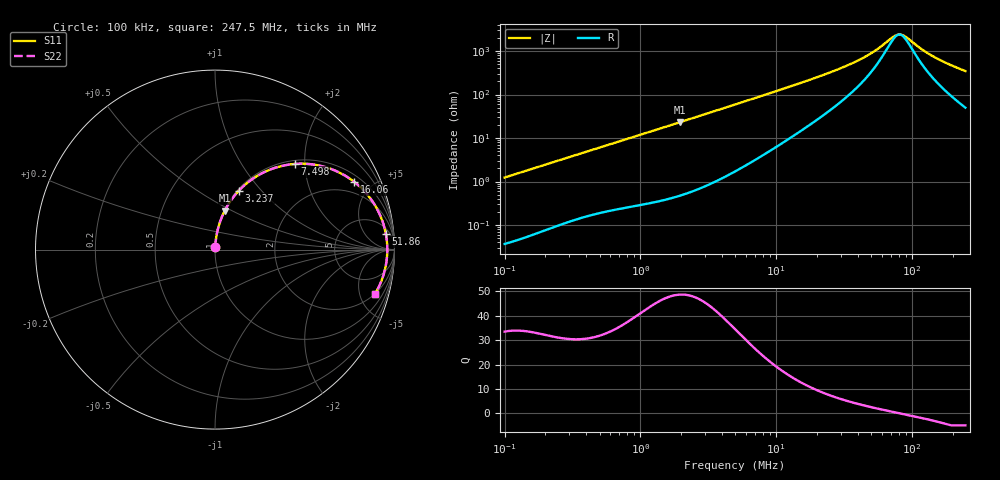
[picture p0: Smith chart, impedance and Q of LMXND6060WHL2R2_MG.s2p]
! LMXND6060WHL2R2_MG  S-PARAMETER MODEL  ( General Type )
! Model Generated by TAIYO YUDEN Corporation (http://www.ty-top.com)
! Version 1.0
! TAIYO YUDEN Control No. 191025NI43SB-FBB
! Copyright(c) 2019 TAIYO YUDEN CO.,LTD. All Rights Reserved.
! Product Description (link to TY-COMPAS)
! https://ds.yuden.co.jp/TYCOMPAS/or/detail?pn=LMXND6060WHL2R2NMG&u=M
! Products Name : Inductors
! Characteristics :
!  Inductance : 2.2 uH , SRF(min) : 68 MHz , DC Resistance(max) : 0.026 Ohm
!  Rated Current : Saturation :4200 mA , Temp Rise : 3700 mA
!  Case Size : 6.0 x 6.0 / 0.236 x 0.236 [mm/inch] , Thickness : 2.8 / 0.11 [mm/inch]
!  (Conditions: Temperature = 25 degC , DC Bias Current/Voltage = 0A / 0V)
! External Node Assignments :
!  1  o---GGG---o  2
! GND o---------o GND
! Frequency Range : 0.1MHz  -  247.502633MHz  [ 402 STEP ]
# MHz S RI R 50
! Freq[MHz].  S11 Real  S11 Imag  S21 Real  S21 Imag  S12 Real  S12 Imag  S22 Real  S22 Imag
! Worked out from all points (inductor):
!   401 points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, 100 kHz to 247.5 MHz, reference 50 ohm
!   read as one part in series: L = 1.97 uH near 104 kHz
!   highest Q = 48.7 at 1.948 MHz (marker M1), where L = 1.88 uH
!   self-resonance near 80.94 MHz
!   S11 on the Smith chart (normalised r, x): 100 kHz: 1.00, +0.02; 3.237 MHz: 1.02, +0.76; 7.498 MHz: 1.07, +1.78; 16.06 MHz: 1.33, +3.92; 51.86 MHz: 9, +17; 247.5 MHz: 2.00, -6.85
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0.1  0.000523 0.0124  0.9995 -0.0124  0.9995 -0.0124  0.000523 0.0124
0.37019  0.00347 0.0446  0.9965 -0.0446  0.9965 -0.0446  0.00347 0.0446
0.76266  0.0106 0.0897  0.9894 -0.0897  0.9894 -0.0897  0.0106 0.0897
1.370406  0.0289 0.157  0.9711 -0.157  0.9711 -0.157  0.0289 0.157
1.947872  0.0544 0.2167  0.9456 -0.2167  0.9456 -0.2167  0.0544 0.2167
3.237002  0.1332 0.3287  0.8668 -0.3287  0.8668 -0.3287  0.1332 0.3287
4.974964  0.2635 0.4263  0.7365 -0.4263  0.7365 -0.4263  0.2635 0.4263
7.498128  0.445 0.4773  0.555 -0.4773  0.555 -0.4773  0.445 0.4773
10.65771  0.6139 0.46  0.3861 -0.46  0.3861 -0.46  0.6139 0.46
16.06301  0.7758 0.3774  0.2242 -0.3774  0.2242 -0.3774  0.7758 0.3774
18.41681  0.8163 0.3419  0.1837 -0.3419  0.1837 -0.3419  0.8163 0.3419
24.68731  0.881 0.2634  0.119 -0.2634  0.119 -0.2634  0.881 0.2634
33.74559  0.9232 0.1839  0.0768 -0.1839  0.0768 -0.1839  0.9232 0.1839
42.66034  0.942 0.1298  0.058 -0.1298  0.058 -0.1298  0.942 0.1298
51.86374  0.9518 0.088  0.0482 -0.088  0.0482 -0.088  0.9518 0.088
68.1772  0.9588 0.0333  0.0412 -0.0333  0.0412 -0.0333  0.9588 0.0333
78.1676  0.9599 0.00673  0.0401 -0.00673  0.0401 -0.00673  0.9599 0.00673
86.18795  0.9598 -0.0121  0.0402 0.0121  0.0402 0.0121  0.9598 -0.0121
117.8121  0.9543 -0.0738  0.0457 0.0738  0.0457 0.0738  0.9543 -0.0738
143.2284  0.9461 -0.1146  0.0539 0.1146  0.0539 0.1146  0.9461 -0.1146
188.2801  0.9263 -0.1767  0.0737 0.1767  0.0737 0.1767  0.9263 -0.1767
247.5026  0.8927 -0.2452  0.1073 0.2452  0.1073 0.2452  0.8927 -0.2452
